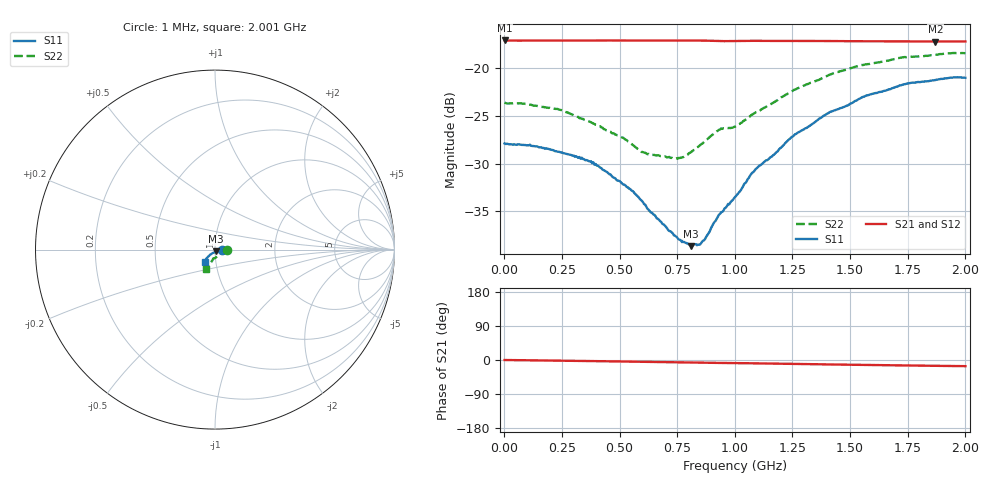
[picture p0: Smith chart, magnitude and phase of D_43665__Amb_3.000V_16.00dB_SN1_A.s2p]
! device id: 43665_
! dir: \\malibu\benchdata\1_engineers\tn_data\43665_75ohm\new\sparar\43665_\amb\3p000v\16p00db
! Serial: 1
! Insertion: A
! Temp: Amb
! VDD: 3.000V
! Attenuation Step: 16.00dB
! IDD: 1.447500e+00mA
! FILE NAME
! DATE 03-27-2009 08:37:17
! CORRECTED  DATA
#  Hz  S  RI  R  75
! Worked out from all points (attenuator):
!   401 points, 1 MHz to 2.001 GHz, reference 75 ohm
!   highest |S21| = -17.07 dB at 1 MHz (marker M1); lowest = -17.2 dB at 1.871 GHz (marker M2)
!   lowest |S11| = -38.7 dB at 811 MHz (marker M3), VSWR 1.02, Z = 75.7 - j1.6 ohm
!   |S11| at or under -10 dB: start of sweep to end of sweep
!   |S22| runs from -29.5 to -18.4 dB; largest |S21 - S12| = 0.00058
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1000000  0.0404 -0.000503  0.1401 -0.000192  0.1403 -0.000176  0.0662 -0.000399
1.21e8  0.0392 6.71e-05  0.1399 -0.00221  0.14 -0.00218  0.0641 -0.000575
2.36e8  0.0365 -0.000522  0.1399 -0.0043  0.1399 -0.00425  0.0608 -0.00232
3.36e8  0.034 -0.0013  0.1398 -0.00617  0.1399 -0.00613  0.0542 -0.00445
4.06e8  0.0309 -0.00137  0.1398 -0.00744  0.1398 -0.00736  0.0495 -0.00684
5.46e8  0.023 -0.00375  0.1396 -0.0104  0.1397 -0.0102  0.0383 -0.0137
6.06e8  0.0188 -0.00477  0.1394 -0.0115  0.1395 -0.0114  0.0319 -0.0171
6.71e8  0.0147 -0.00656  0.1394 -0.0128  0.1395 -0.0127  0.0272 -0.022
7.46e8  0.00964 -0.00887  0.1393 -0.0145  0.1394 -0.0143  0.0202 -0.0271
8.11e8  0.00502 -0.0105  0.1391 -0.016  0.1391 -0.0158  0.0137 -0.0338
8.61e8  0.00104 -0.0124  0.1388 -0.0172  0.1388 -0.017  0.009 -0.0395
9.31e8  -0.00525 -0.0162  0.1379 -0.0187  0.1381 -0.0184  -0.000453 -0.0476
1.001e9  -0.0105 -0.0183  0.1378 -0.0194  0.138 -0.0191  -0.00903 -0.0486
1.096e9  -0.0188 -0.0233  0.1377 -0.0217  0.1379 -0.0214  -0.0134 -0.0574
1.251e9  -0.0301 -0.0319  0.1371 -0.0249  0.1374 -0.0245  -0.0227 -0.0728
1.336e9  -0.0355 -0.0367  0.1367 -0.0265  0.1371 -0.0263  -0.0278 -0.0799
1.411e9  -0.0408 -0.0424  0.1362 -0.0284  0.1366 -0.0282  -0.0301 -0.0876
1.561e9  -0.0488 -0.0516  0.1353 -0.0311  0.1358 -0.0311  -0.0381 -0.0973
1.671e9  -0.0528 -0.0571  0.1346 -0.0332  0.135 -0.0332  -0.0422 -0.1018
1.756e9  -0.055 -0.0629  0.1341 -0.0347  0.1346 -0.0349  -0.0446 -0.1058
1.871e9  -0.0562 -0.0662  0.1334 -0.0366  0.1335 -0.0366  -0.0488 -0.1074
2.001e9  -0.056 -0.0695  0.1329 -0.0387  0.1328 -0.039  -0.0517 -0.1085
